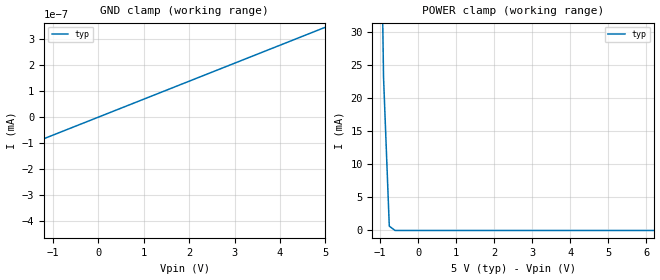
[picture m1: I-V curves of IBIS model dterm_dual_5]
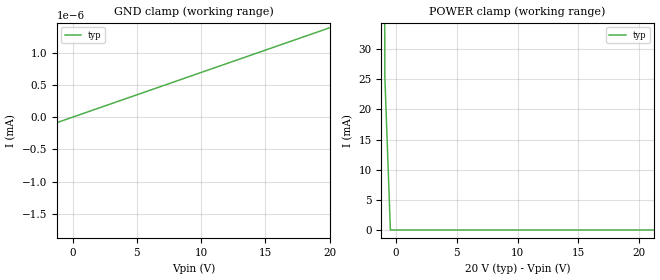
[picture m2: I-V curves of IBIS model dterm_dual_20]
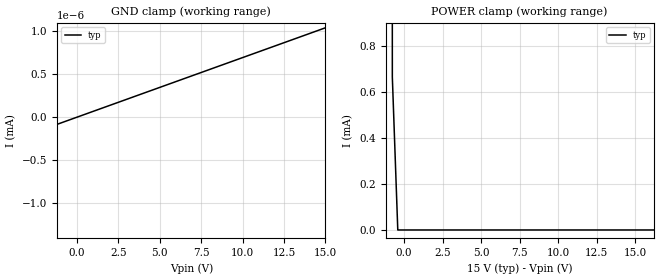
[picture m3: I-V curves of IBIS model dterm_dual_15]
|Texas Instruments Incorporated
|tmux7221, 2 Data Lane 1:1 44V Precision mux
[IBIS Ver]   4.1
[File name]   tmux7221.ibs
[Date]   12/01/22
[File Rev]   1.0
[Source]
| Texas Instruments Incorporated.
| ASC-INT-MPD
| 12500 TI Blvd
| Dallas, TX - 75243
[Notes]   Revision History:
| Rev 1.0: 12/01/22
| - Initial version of the model
| - Model generated from simulations in SPECTRE
| - C_comp although listed in numerical order of value are
|   obtained from varying PVT conditions. For PVT conditions for
|   each specific value refer the buffer description under
|   respective [Model]. IBIS model user is responsible for using
|   appropriate C_comp to simulate for Signal Integrity.
[Disclaimer]
| This model is designed as an aid for customers of Texas Instruments.
| TI and its licensors and suppliers make no warranties, either expressed
| or implied, with respect to this  model, including the warranties of
| merchantability or fitness for a particular purpose. The model is
| provided solely on an "as is" basis. The entire risk as to its quality
| and performance is with the customer.
| This model is subject to change without notice. Texas Instruments
| Incorporated is not responsible for updating this model.
[Copyright]
(C) Copyright 2022 Texas Instruments Incorporated.All rights reserved.
|  Component TMUX7221DGS 10-pin - DGS package
|  Part # TMUX7221DGS
[Component]   TMUX7221DGS
[Manufacturer]  TI
[Package]
|   typ   min   max
R_pkg   0.0668   NA   NA
L_pkg   2.1992nH   NA   NA
C_pkg   0.2884pF   NA   NA
[Pin]   signal_name   model_name
   1   S1   sterm
   2   S2   sterm
   3   NC   nc
   4   GND   gnd
   5   VDD   power
   6   SEL2   inbuf
   7   SEL1   inbuf
   8   VSS   power
   9   D2   dterm
   10   D1   dterm
[Series Switch Groups]
On 1 /
On 2 /
Off 1 2 /
[Series Pin Mapping]  pin_2 model_name function_table_group
   1  10   switch_dual_5   1
   2   9   switch_dual_5   1
|   1  10   switch_dual_20   1
|   2   9   switch_dual_20   1
|   1  10   switch_dual_15   1
|   2   9   switch_dual_15   1
|   1  10   switch_36   1
|   2   9   switch_36   1
|   1  10   switch_44   1
|   2   9   switch_44   1
|   1  10   switch_12   1
|   2   9   switch_12   1
|  Component TMUX7221DSC 10-pin - DSC package
|  Part # TMUX7221DSC
[Component]   TMUX7221DSC
[Manufacturer]  TI
[Package]
|   typ   min   max
R_pkg   0.0668   NA   NA
L_pkg   2.1992nH   NA   NA
C_pkg   0.2884pF   NA   NA
[Pin]   signal_name   model_name
   1   S1   sterm
   2   S2   sterm
   3   NC   nc
   4   GND   gnd
   5   VDD   power
   6   SEL2   inbuf
   7   SEL1   inbuf
   8   VSS   power
   9   D2   dterm
   10   D1   dterm
[Series Switch Groups]
On 1 /
On 2 /
Off 1 2 /
[Series Pin Mapping]  pin_2 model_name function_table_group
|   1  10   switch_dual_5   1
|   2   9   switch_dual_5   1
|   1  10   switch_dual_20   1
|   2   9   switch_dual_20   1
|   1  10   switch_dual_15   1
|   2   9   switch_dual_15   1
|   1  10   switch_36   1
|   2   9   switch_36   1
|   1  10   switch_44   1
|   2   9   switch_44   1
   1  10   switch_12   1
   2   9   switch_12   1
[Model Selector] dterm
dterm_dual_5 Use for operation at +/-5V
dterm_dual_20 Use for operation at +/-20V
dterm_dual_15 Use for operation at +/-15V
dterm_36 Use for operation at 36V
dterm_44 Use for operation at 44V
dterm_12 Use for operation at 12V
[Model Selector] sterm
sterm_dual_5 Use for operation at +/-5V
sterm_dual_20 Use for operation at +/-20V
sterm_dual_15 Use for operation at +/-15V
sterm_36 Use for operation at 36V
sterm_44 Use for operation at 44V
sterm_12 Use for operation at 12V
[Model Selector] inbuf
inbuf_dual_5 Use for operation at +/-5V
inbuf_dual_20 Use for operation at +/-20V
inbuf_dual_15 Use for operation at +/-15V
inbuf_36 Use for operation at 36V
inbuf_44 Use for operation at 44V
inbuf_12 Use for operation at 12V
| switch_dual_5
[Model]   switch_dual_5
Model_type   Series_switch
|   typ   min   max
C_comp   1.008417e-11   NA   NA
[Voltage Range]   5   NA   NA
[Power Clamp Reference]   5   NA   NA
[Temperature Range]   27   NA   NA
[On]
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[Off]
|   typ   min   max
[R Series]   10G   NA   NA
| switch_dual_20
[Model]   switch_dual_20
Model_type   Series_switch
|   typ   min   max
C_comp   1.598234e-11   NA   NA
[Voltage Range]   20   NA   NA
[Power Clamp Reference]   20   NA   NA
[Temperature Range]   27   NA   NA
[On]
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[Off]
|   typ   min   max
[R Series]   10G   NA   NA
| switch_dual_15
[Model]   switch_dual_15
Model_type   Series_switch
|   typ   min   max
C_comp   1.598234e-11   NA   NA
[Voltage Range]   15   NA   NA
[Power Clamp Reference]   15   NA   NA
[Temperature Range]   27   NA   NA
[On]
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[Off]
|   typ   min   max
[R Series]   10G   NA   NA
| switch_36
[Model]   switch_36
Model_type   Series_switch
|   typ   min   max
C_comp   1.598234e-11   NA   NA
[Voltage Range]   36   NA   NA
[Power Clamp Reference]   36   NA   NA
[Temperature Range]   27   NA   NA
[On]
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[Off]
|   typ   min   max
[R Series]   10G   NA   NA
| switch_44
[Model]   switch_44
Model_type   Series_switch
|   typ   min   max
C_comp   1.598234e-11   NA   NA
[Voltage Range]   44   NA   NA
[Power Clamp Reference]   44   NA   NA
[Temperature Range]   27   NA   NA
[On]
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[Off]
|   typ   min   max
[R Series]   10G   NA   NA
| switch_12
[Model]   switch_12
Model_type   Series_switch
|   typ   min   max
C_comp   1.008417e-11   NA   NA
[Voltage Range]   12   NA   NA
[Power Clamp Reference]   12   NA   NA
[Temperature Range]   27   NA   NA
[On]
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[Off]
|   typ   min   max
[R Series]   10G   NA   NA
| Models and submodels in the file (24): dterm_dual_5 (Terminator), dterm_dual_20 (Terminator), dterm_dual_15 (Terminator), dterm_36 (Terminator), dterm_44 (Terminator), dterm_12 (Terminator), switch_dual_5 (Series_switch), switch_dual_20 (Series_switch), switch_dual_15 (Series_switch), switch_36 (Series_switch), switch_44 (Series_switch), switch_12 (Series_switch), sterm_dual_5 (Terminator), sterm_dual_20 (Terminator), sterm_dual_15 (Terminator), sterm_36 (Terminator), sterm_44 (Terminator), sterm_12 (Terminator), inbuf_dual_5 (Input), inbuf_dual_20 (Input), inbuf_dual_15 (Input), inbuf_36 (Input), inbuf_44 (Input), inbuf_12 (Input)
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| dterm_dual_5
[Model]   dterm_dual_5
Model_type   Terminator
|   typ   min   max
C_comp   1.008417e-11   NA   NA
[Voltage Range]   5   NA   NA
[Temperature Range]   27   NA   NA
[Power Clamp Reference]   5   NA   NA
[GND Clamp Reference]   0   NA   NA
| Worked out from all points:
|   GND clamp passes 1 mA (typ) near -5.76 V on its own axis
|   POWER clamp passes 1 mA (typ) near -0.76 V on its own axis
[GND Clamp]
|   Voltage   I(typ)   I(min)   I(max)
-10V      -4.767A    NA         NA
-5.303V   -553.8pA   NA         NA
-5.152V   -360.1pA   NA         NA
-5V       -347pA     NA         NA
5V        346.8pA    NA         NA
[POWER Clamp]
|   Voltage   I(typ)   I(min)   I(max)
-5V       5.369A     NA         NA
-1.061V   84.43mA    NA         NA
-909.1mV  23.3mA     NA         NA
-757.6mV  659.6uA    NA         NA
-606.1mV  3.286uA    NA         NA
10V       -347pA     NA         NA
| dterm_dual_20
[Model]   dterm_dual_20
Model_type   Terminator
|   typ   min   max
C_comp   1.598234e-11   NA   NA
[Voltage Range]   20   NA   NA
[Temperature Range]   27   NA   NA
[Power Clamp Reference]   20   NA   NA
[GND Clamp Reference]   0   NA   NA
[GND Clamp]
|   Voltage   I(typ)   I(min)   I(max)
-25V      -4.884A    NA         NA
-20.45V   -21.91nA   NA         NA
-20V      -1.383nA   NA         NA
20V       1.383nA    NA         NA
[POWER Clamp]
|   Voltage   I(typ)   I(min)   I(max)
-5V       5.383A     NA         NA
-1.364V   353.7mA    NA         NA
-909.1mV  25.39mA    NA         NA
-454.5mV  16.97nA    NA         NA
40V       -1.383nA   NA         NA
| dterm_dual_15
[Model]   dterm_dual_15
Model_type   Terminator
|   typ   min   max
C_comp   1.598234e-11   NA   NA
[Voltage Range]   15   NA   NA
[Temperature Range]   27   NA   NA
[Power Clamp Reference]   15   NA   NA
[GND Clamp Reference]   0   NA   NA
[GND Clamp]
|   Voltage   I(typ)   I(min)   I(max)
-20V      -4.859A    NA         NA
-15.4V    -5.116nA   NA         NA
-15.05V   -1.042nA   NA         NA
15V       1.038nA    NA         NA
[POWER Clamp]
|   Voltage   I(typ)   I(min)   I(max)
-5V       5.38A      NA         NA
-1.111V   123.1mA    NA         NA
-757.6mV  666.4uA    NA         NA
-404mV    3.734nA    NA         NA
30V       -1.038nA   NA         NA
